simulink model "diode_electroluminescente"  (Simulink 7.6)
settings: Solver=ode15s  StartTime=0.0  StopTime=1.0  RelTol=1e-3
StopFcn:
  | load signaux.mat
  | plot(x(1,:),x(2,:),x(1,:),x(3,:))
  | title('Dérivateur commandé par PWL Current et source I-->V')
  | xlabel('temps')
  | axis([0 1 -0.6 1.2]), grid
  | gtext('Tension d''entrée')
  | gtext('Sortie dela diode')
undefined symbols (not defined in the file or in its folder): sigbuilder_block
libraries: fl_lib x6, nesl_utility x4, elec_lib x2

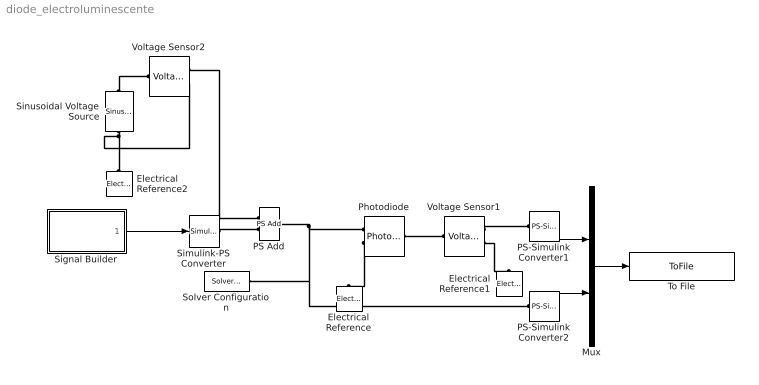
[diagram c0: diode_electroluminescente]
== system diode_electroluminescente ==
  Electrical Reference : fl_lib/Electrical/Electrical Elements/Electrical Reference  DialogController=NetworkEngine.DynNeDlgSource  SystemSampleTime=-1  i_Log=off  LocalVarNames=|i  LocalVarDescs=|i  LocalVarLogging=[]
  Electrical Reference1 : fl_lib/Electrical/Electrical Elements/Electrical Reference  DialogController=NetworkEngine.DynNeDlgSource  SystemSampleTime=-1  i_Log=off  LocalVarNames=|i  LocalVarDescs=|i  LocalVarLogging=[]
  Electrical Reference2 : fl_lib/Electrical/Electrical Elements/Electrical Reference  DialogController=NetworkEngine.DynNeDlgSource  SystemSampleTime=-1  i_Log=off  LocalVarNames=|i  LocalVarDescs=|i  LocalVarLogging=[]
  Mux : Mux  Inputs=2
  PS Add : fl_lib/Physical Signals/Functions/PS Add  DialogController=NetworkEngine.DynNeDlgSource  SystemSampleTime=-1  LocalVarLogging=[]
  PS-Simulink Converter1 : nesl_utility/PS-Simulink Converter  DialogController=NetworkEngine.DynNeUtilDlgSource  SystemSampleTime=-1  PhysicalDomain=network_engine_domain  LeftPortType=input  RightPortType=output  SubClassName=ps_output  Unit=V  AffineConversion=off
  PS-Simulink Converter2 : nesl_utility/PS-Simulink Converter  DialogController=NetworkEngine.DynNeUtilDlgSource  SystemSampleTime=-1  PhysicalDomain=network_engine_domain  LeftPortType=input  RightPortType=output  SubClassName=ps_output  Unit=V  AffineConversion=off
  Photodiode : elec_lib/Sensors/Photodiode  DialogController=NetworkEngine.DynNeDlgSource  SystemSampleTime=-1  prmFlux=1  Imeas=25 uA  FluxD=5 W/m^2  G=5e-06 m^2*A/W  prmExp=1  I2=0.08 A  V2=1.3 V  RS=0.1 Ohm  IS=5e-09 A  Tmeas=25 C  ec=3  C_param=1  CJ0=60 pF  VJ=1 V  Mgrad=0.5  Vvec="[  0.1 10 100 ] V"  Cvec="[  45 30 6 ] pF"  FC=0.5  LocalVarLogging=[]
  Signal Builder : Subsystem  Tag=STV Subsys  LoadFcn=sigbuilder_block('load');  StartFcn=sigbuilder_block('start');  StopFcn=sigbuilder_block('stop');  ClipboardFcn=sigbuilder_block('clipboard');
  Simulink-PS Converter : nesl_utility/Simulink-PS Converter  DialogController=NetworkEngine.DynNeUtilDlgSource  SystemSampleTime=-1  PhysicalDomain=network_engine_domain  LeftPortType=input  RightPortType=output  SubClassName=ps_input  Unit=1  AffineConversion=off  InputFilterTimeConstant=.001  UdotUserProvided=0
  Sinusoidal Voltage Source : elec_lib/Additional Components/SPICE-Compatible Components/Sources/Sinusoidal Voltage Source  DialogController=NetworkEngine.DynNeDlgSource  SystemSampleTime=-1  VO=0 V  VA=20 mV  FREQ=10 Hz  TD=0 s  DF=0 1/s  current_Log=off  voltage_Log=off  power_Log=off  LocalVarNames=|current|voltage|power  LocalVarDescs=|Current (A)|Voltage (V)|Power (W)  LocalVarLogging=[0 0 0]
  Solver Configuration : nesl_utility/Solver Configuration  DialogController=NetworkEngine.DynNeUtilDlgSource  SystemSampleTime=-1  PhysicalDomain=network_engine_domain  LeftPortType=input  RightPortType=generic  SubClassName=solver  Accelerate=off  Profile=off  ResidualTolerance=1e-9  MaxNonlinIter=12  MaxModeIter=2  DoFixedCost=off  UseLocalSampling=off  DoDC=off  LinearAlgebra=Sparse  LocalSolverSampleTime=.001  LocalSolverChoice=NE_BACKWARD_EULER_ADVANCER  UseLocalSolver=off
  To File : ToFile  Filename=signaux  MatrixName=x
  Voltage Sensor1 : fl_lib/Electrical/Electrical Sensors/Voltage Sensor  DialogController=NetworkEngine.DynNeDlgSource  SystemSampleTime=-1  i1_Log=off  v1_Log=off  LocalVarNames=|i1|v1  LocalVarDescs=|i1|v1  LocalVarLogging=[]
  Voltage Sensor2 : fl_lib/Electrical/Electrical Sensors/Voltage Sensor  DialogController=NetworkEngine.DynNeDlgSource  SystemSampleTime=-1  i1_Log=off  v1_Log=off  LocalVarNames=|i1|v1  LocalVarDescs=|i1|v1  LocalVarLogging=[]
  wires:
  Signal Builder/1(Signal 2) -> Simulink-PS Converter/1
  PS-Simulink Converter1/1 -> Mux/1
  Mux/1 -> To File/1
  PS-Simulink Converter2/1 -> Mux/2
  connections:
  Solver Configuration/RConn1 -- Photodiode/LConn1 -- PS Add/RConn1 -- PS-Simulink Converter2/LConn1
  Photodiode/LConn2 -- Electrical Reference/LConn1
  Photodiode/RConn1 -- Voltage Sensor1/LConn1
  Voltage Sensor1/RConn1 -- PS-Simulink Converter1/LConn1
  Voltage Sensor1/RConn2 -- Electrical Reference1/LConn1
  Simulink-PS Converter/RConn1 -- PS Add/LConn2
  Sinusoidal Voltage Source/RConn1 -- Electrical Reference2/LConn1 -- Voltage Sensor2/RConn2
  Sinusoidal Voltage Source/LConn1 -- Voltage Sensor2/LConn1
  Voltage Sensor2/RConn1 -- PS Add/LConn1

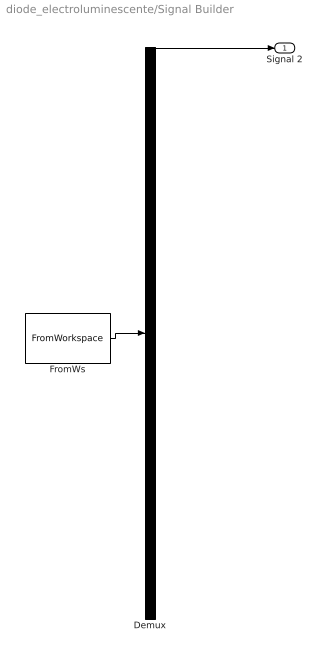
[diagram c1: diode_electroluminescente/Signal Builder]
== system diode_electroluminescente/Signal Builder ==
  Demux : Demux  Tag=STV Demux  Outputs=1
  FromWs : FromWorkspace  Tag=STV FromWs  VariableName=tuvar  SampleTime=0  SigBuilderData=DataTag0  VnvData=DataTag1
  Signal 2 : Outport  Tag=STV Outport
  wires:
  Demux/1 -> Signal 2/1
  FromWs/1 -> Demux/1
